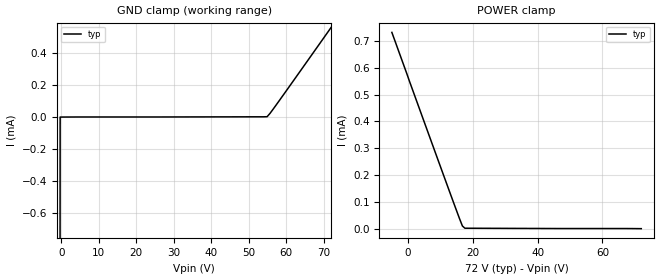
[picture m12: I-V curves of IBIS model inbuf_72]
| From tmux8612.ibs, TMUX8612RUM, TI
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| inbuf_72
[Model]   inbuf_72
Model_type   Input
Vinl = 0.8
Vinh = 1.3
|   typ   min   max
C_comp   6.362683e-13   NA   NA
[Voltage Range]   72   NA   NA
[Temperature Range]   27   NA   NA
[Power Clamp Reference]   72   NA   NA
[GND Clamp Reference]   0   NA   NA
[GND Clamp]
|   Voltage   I(typ)   I(min)   I(max)
-5V       -911.1mA   NA         NA
-1.111V   -26.3mA    NA         NA
-333.3mV  -231.8nA   NA         NA
54.89V    2.206uA    NA         NA
58V       98.78uA    NA         NA
72V       563.9uA    NA         NA
[POWER Clamp]
|   Voltage   I(typ)   I(min)   I(max)
-5V       731.6uA    NA         NA
15.22V    58.81uA    NA         NA
16.78V    9.908uA    NA         NA
17.56V    1.614uA    NA         NA
72V       -139.7pA   NA         NA
